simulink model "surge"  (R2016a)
settings: Solver=ode5  StartTime=0.0  StopTime=60.0  FixedStep=0.001  RelTol=1e-3
undefined symbols (not defined in the file): gain, initialv, initialy, K_cd, K_p, meansurgeerror, reactiontime, surgethreshold, T_I, T_L, T_N, target, tau, tau2

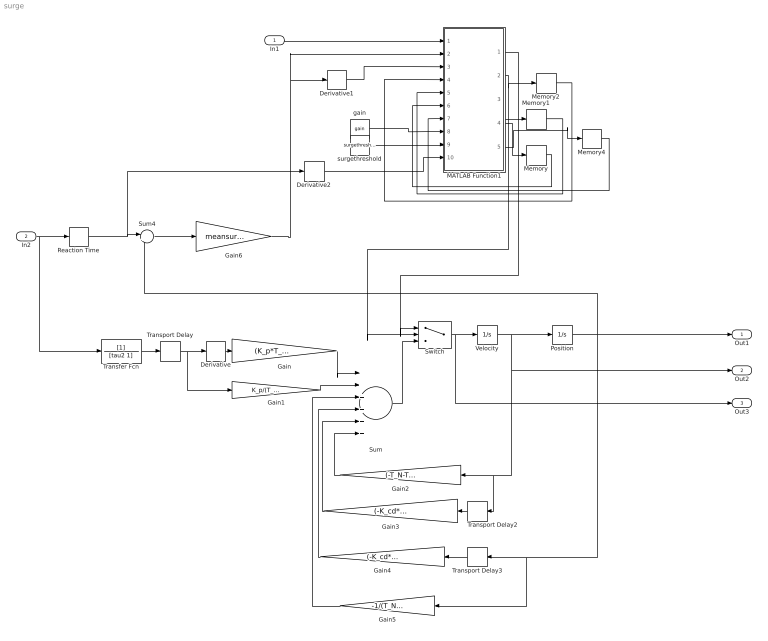
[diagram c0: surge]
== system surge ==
  In1 : Inport
  In2 : Inport  Port=2
  Derivative : Derivative
  Derivative1 : Derivative
  Derivative2 : Derivative
  Gain : Gain  Gain=(K_p*T_L)/(T_N*T_I)
  Gain1 : Gain  Gain=K_p/(T_N*T_I)
  Gain2 : Gain  Gain=(-T_N-T_I)/(T_N*T_I)
  Gain3 : Gain  Gain=(-K_cd*K_p*T_L)/(T_N*T_I)
  Gain4 : Gain  Gain=(-K_cd*K_p)/(T_N*T_I)
  Gain5 : Gain  Gain=-1/(T_N*T_I)
  Gain6 : Gain  Gain=meansurgeerror
  MATLAB Function1 : MATLAB Function  TreatAsAtomicUnit=on
  Memory{,1..2,4} (4 alike) : Memory
  Position : Integrator  InitialCondition=initialy
  Reaction Time : TransportDelay  DelayTime=reactiontime  InitialOutput=target(1)
  Sum : Sum  Inputs=|++++++
  Sum4 : Sum  Inputs=|+-
  Switch : Switch  Criteria=u2 ~= 0
  Transfer Fcn : TransferFcn  Denominator=[tau2 1]
  Transport Delay : TransportDelay  DelayTime=tau
  Transport Delay2 : TransportDelay  DelayTime=tau
  Transport Delay3 : TransportDelay  DelayTime=tau
  Velocity : Integrator  InitialCondition=initialv
  gain : Constant  Value=gain
  surgethreshold : Constant  Value=surgethreshold
  Out1 : Outport
  Out2 : Outport  Port=2
  Out3 : Outport  Port=3
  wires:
  In1/1 -> MATLAB Function1/1(time)
  MATLAB Function1/4(newtswitch) -> Memory/1
  Memory/1 -> MATLAB Function1/6(tswitch)
  MATLAB Function1/3(newt0) -> Memory1/1
  Memory1/1 -> MATLAB Function1/5(t0)
  MATLAB Function1/2(newlocked) -> Switch/2, Memory2/1
  Memory2/1 -> MATLAB Function1/4(locked)
  MATLAB Function1/1(aout) -> Switch/1
  gain/1 -> MATLAB Function1/8(a_max)
  surgethreshold/1 -> MATLAB Function1/9(surgethreshold)
  Gain6/1 -> Derivative1/1, MATLAB Function1/2(e)
  Velocity/1 -> Position/1, Gain2/1, Transport Delay2/1, Out2/1
  Transport Delay/1 -> Gain1/1, Derivative/1
  Derivative/1 -> Gain/1
  Gain/1 -> Sum/1
  Gain1/1 -> Sum/2
  Gain2/1 -> Sum/6
  Transport Delay2/1 -> Gain3/1
  Gain3/1 -> Sum/5
  Transport Delay3/1 -> Gain4/1
  Gain4/1 -> Sum/4
  Gain5/1 -> Sum/3
  Sum/1 -> Switch/3
  Switch/1 -> Out3/1, Velocity/1
  Position/1 -> Out1/1, Gain5/1, Transport Delay3/1, Sum4/2
  Transfer Fcn/1 -> Transport Delay/1
  MATLAB Function1/5(newtstop) -> Memory4/1
  Memory4/1 -> MATLAB Function1/7(tstop)
  Derivative1/1 -> MATLAB Function1/3(edot)
  Derivative2/1 -> MATLAB Function1/10(tdot)
  In2/1 -> Transfer Fcn/1, Reaction Time/1
  Sum4/1 -> Gain6/1
  Reaction Time/1 -> Derivative2/1, Sum4/1

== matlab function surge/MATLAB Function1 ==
function [aout,newlocked, newt0, newtswitch, newtstop]  = fcn(time,e, edot, locked,t0,tswitch, tstop, a_max, surgethreshold, tdot)
newt0 = t0;
newtswitch = tswitch;
newtstop = tstop;
newlocked = locked;
aout=0;%k1*e; % activate local control law if no other conditions met

a_1 = 1.0;      % constant for abs error weight
a_2 = 0.01;     % constant for abs error derivative weight

if locked ~= 0 
    if time-t0 < tswitch 
       aout = locked*a_max; % first bang
    elseif time-t0 < tstop
       aout = -locked*a_max; % second bang
    else
       newlocked = 0;       % end of bang-bang. Unlock
    end
elseif (a_1*abs(e)+a_2*abs(edot) > surgethreshold && abs(tdot)<1) %&& abs(wait-e)<10          % threshold below which surge model is used
    %we must not execute a bang WHILE the target is changing, because
    %otherwise we hopelessly overshoot because edot is infinite during the
    %target switch. As a hack, bang only when abs(edot)<100.
    if e == -edot*abs(edot)/(2*a_max)
        f0 = sign(edot);                            % eqn (11)
    else
        f0 = sign(edot*abs(edot)/(2*a_max) + e);    % eqn (9) & (10) of Costello
    end
  %  if f0 == sign(edot) % eqn (13) in Costello doesn't really make sense -
                         %  would need to set a flag that e == -edot*abs(edot)/(2*a_max)
   %     newtswitch = 0;
  % else
        
        newtswitch = sqrt(0.5*(edot/(a_max*f0)).^2+ e/(a_max*f0)) ...
                     + edot/(a_max*f0); % eqn (12) from Costello
   % end
        
    newlocked = f0;    % lock, and give information about direction of error which is fed back
    
    newt0=time;             % remember start of bang-bang 
    newtstop = newtswitch + sqrt(0.5*(edot/(a_max*f0)).^2 + e/(a_max*f0)); %
    aout = newlocked*a_max;
end
